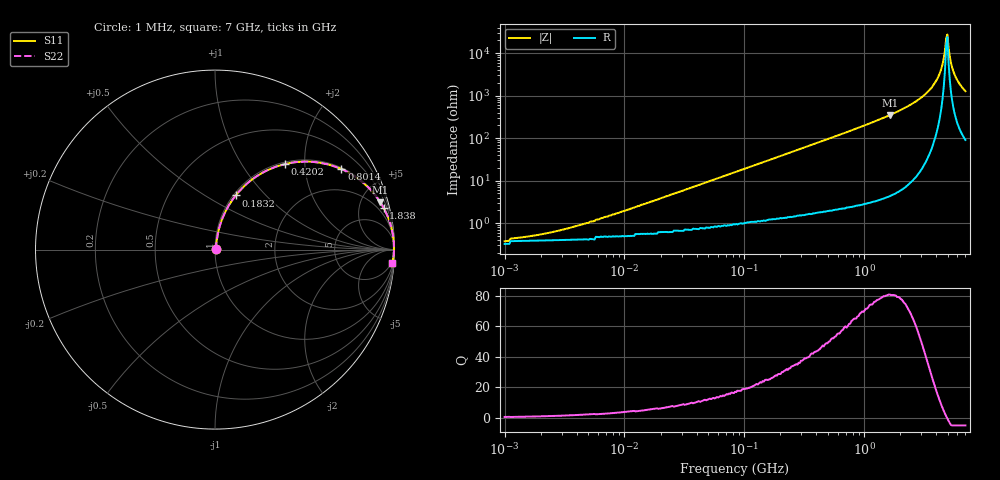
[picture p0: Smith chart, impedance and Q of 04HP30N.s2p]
# MHz S MA R 50
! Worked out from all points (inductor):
!   385 points, 1 MHz to 7 GHz, reference 50 ohm
!   read as one part in series: L = 29.9 nH near 7.784 MHz
!   highest Q = 80.5 at 1.638 GHz (marker M1), where L = 33.7 nH
!   self-resonance near 4.84 GHz
!   S11 on the Smith chart (normalised r, x): 1 MHz: 1.01, +0.00; 183.2 MHz: 1.03, +0.69; 420.2 MHz: 1.04, +1.60; 801.4 MHz: 1.05, +3.11; 1.838 GHz: 1.09, +8.06; 7 GHz: 3, -25
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1  0.003935 28.4  0.997 -0.1  0.997 -0.1  0.003935 28.4
2.044  0.005376 45.3  0.996 -0.2  0.996 -0.2  0.005376 45.3
4.374  0.009238 62.2  0.996 -0.5  0.996 -0.5  0.009238 62.2
19.575  0.037 78.8  0.993 -2.1  0.993 -2.1  0.037 78.8
85.617  0.158 77.6  0.978 -9.1  0.978 -9.1  0.158 77.6
183.232  0.323 69.1  0.935 -18.9  0.935 -18.9  0.323 69.1
365.931  0.564 54.3  0.813 -34.3  0.813 -34.3  0.564 54.3
420.222  0.617 50.6  0.773 -38.1  0.773 -38.1  0.617 50.6
801.401  0.835 32.5  0.538 -56.6  0.538 -56.6  0.835 32.5
1637.803  0.958 16.0  0.276 -73.3  0.276 -73.3  0.958 16.0
1837.926  0.968 13.9  0.24 -75.4  0.24 -75.4  0.968 13.9
2914.698  0.991 6.7  0.117 -82.2  0.117 -82.2  0.991 6.7
3843.73  0.996 3.1  0.053 -84.3  0.053 -84.3  0.996 3.1
4414.002  0.997 1.3  0.023 -81.9  0.023 -81.9  0.997 1.3
4730.122  0.997 0.5  0.008694 -69.4  0.008694 -69.4  0.997 0.5
4840.449  0.997 0.2  0.004443 -45.9  0.004443 -45.9  0.997 0.2
4953.349  0.997 -0.1  0.003636 28.9  0.003636 28.9  0.997 -0.1
5068.882  0.997 -0.4  0.007481 63.6  0.007481 63.6  0.997 -0.4
5187.11  0.997 -0.7  0.012 73.1  0.012 73.1  0.997 -0.7
5558.598  0.996 -1.5  0.027 80.4  0.027 80.4  0.996 -1.5
6095.627  0.995 -2.7  0.047 82.0  0.047 82.0  0.995 -2.7
7000  0.991 -4.4  0.078 81.5  0.078 81.5  0.991 -4.4
